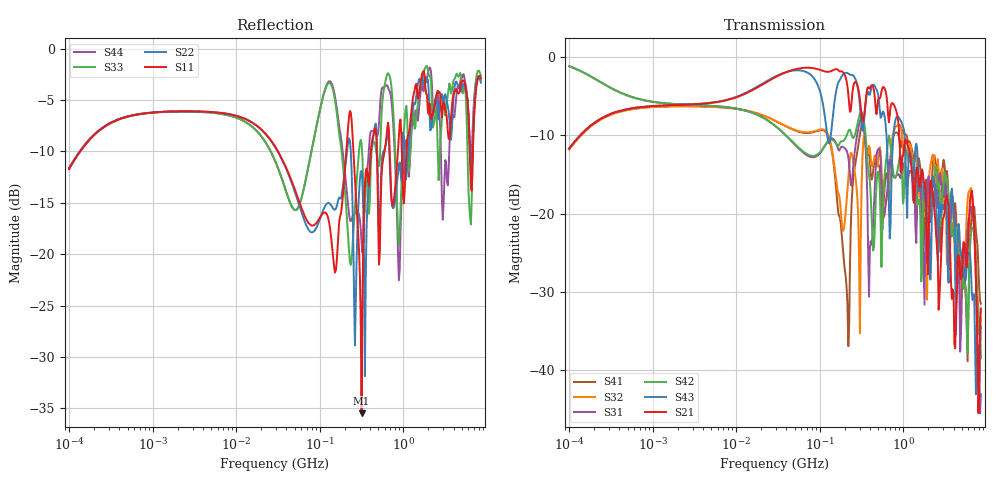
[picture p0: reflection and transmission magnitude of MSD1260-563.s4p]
# MHz S MA R 50
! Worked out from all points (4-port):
!   498 points, 100 kHz to 8.5 GHz, reference 50 ohm
!   strongest paths, dB at 100 kHz, 1.698 MHz, 29.49 MHz, 500.7 MHz, 8.5 GHz:
!     S21: -11.7, -6.1, -2.5, -5.4, -32.2
!     S43: -11.7, -6.1, -2.4, -4.8, -34.4
!     S42: -1.1, -5.9, -8.8, -14.6, -38.5
!     S31: -1.1, -5.9, -8.8, -11.8, -43.1
!     S32: -11.8, -6.3, -8.1, -13.3, -33.4
!     S41: -11.8, -6.3, -8.1, -13.9, -31.5
!   lowest |S11| = -35.5 dB at 317.1 MHz (marker M1), VSWR 1.03, Z = 51.7 - j0.245 ohm
!   |S11| at or under -10 dB: 31.67 MHz to 208 MHz (176.3 MHz wide, 147 % of centre); 688.2 MHz to 863.8 MHz (175.6 MHz wide, 22.6 % of centre); 6.266 GHz to 6.83 GHz (564.1 MHz wide, 8.62 % of centre)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
0.1  0.2594 56.6  0.261 57.1  0.8785 -14.5  0.2579 -123.5
     0.261 57.1  0.2608 56.3  0.2582 -123.5  0.8771 -14.6
     0.8785 -14.5  0.2582 -123.5  0.2602 56.5  0.2605 56.9
     0.2579 -123.5  0.8771 -14.6  0.2605 56.9  0.2613 56.2
113.4622  0.1593 -18.2  0.8143 -23.3  0.2682 163.8  0.3393 14.6
          0.8143 -23.3  0.1683 -7.5  0.3441 19.2  0.2682 176.2
          0.2682 163.8  0.3441 19.2  0.611 -6.4  0.4447 -49.0
          0.3393 14.6  0.2682 176.2  0.4447 -49.0  0.6163 1.7
215.0626  0.3801 14.8  0.6491 -63.1  0.2442 18.1  0.02537 -3.8
          0.6491 -63.1  0.3316 -24.6  0.1454 34.4  0.3264 52.8
          0.2442 18.1  0.1454 34.4  0.1357 -141.1  0.7933 -36.6
          0.02537 -3.8  0.3264 52.8  0.7933 -36.6  0.1853 -77.3
317.0858  0.01684 -8.1  0.4293 -68.8  0.4079 -41.4  0.3682 16.3
          0.4293 -68.8  0.2534 -21.8  0.1479 74.3  0.4457 -30.2
          0.4079 -41.4  0.1479 74.3  0.3452 -12.7  0.3627 -72.5
          0.3682 16.3  0.4457 -30.2  0.3627 -72.5  0.1135 -131.7
1970.81  0.4986 178.1  0.04087 124.3  0.1637 -167.5  0.1297 160.1
         0.04087 124.3  0.706 179.5  0.05982 -130.1  0.0963 158.8
         0.1637 -167.5  0.05982 -130.1  0.7816 -175.0  0.1017 106.0
         0.1297 160.1  0.0963 158.8  0.1017 106.0  0.7594 -164.3
6611.76  0.2031 88.8  0.1402 12.2  0.1062 50.6  0.09931 113.8
         0.1402 12.2  0.2605 107.5  0.1371 59.3  0.08101 87.1
         0.1062 50.6  0.1371 59.3  0.1904 101.8  0.03126 -40.6
         0.09931 113.8  0.08101 87.1  0.03126 -40.6  0.3039 96.6
8500  0.7194 -56.7  0.02467 -15.8  0.006986 -45.3  0.0265 -121.2
      0.02467 -15.8  0.6819 -58.5  0.02127 -108.0  0.01185 -108.7
      0.006986 -45.3  0.02127 -108.0  0.74 -52.8  0.01906 15.7
      0.0265 -121.2  0.01185 -108.7  0.01906 15.7  0.7049 -56.5
